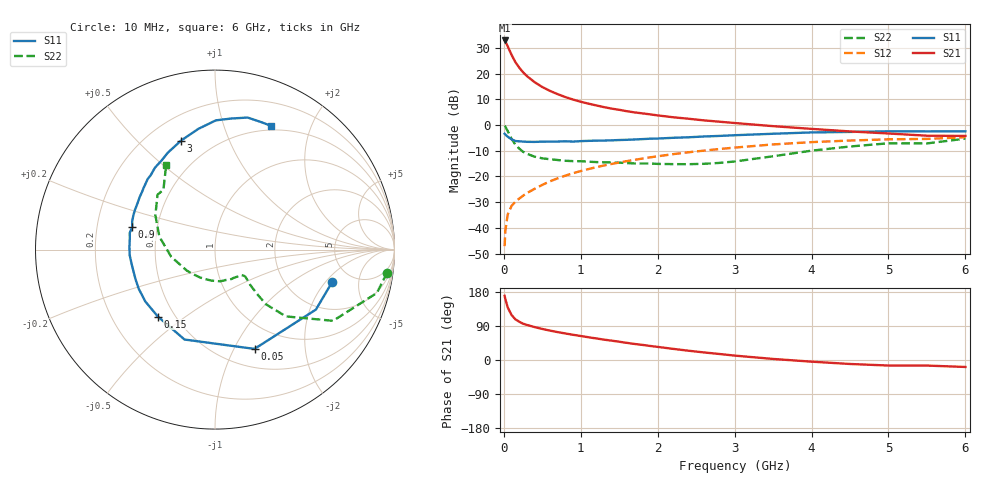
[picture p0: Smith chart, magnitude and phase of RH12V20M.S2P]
! SIEMENS Small Signal Semiconductors
! BFR106
! Si NPN RF Bipolar Junction Transistor in SOT23
! VCE = 12 V  IC = 20 mA
! Common Emitter S-Parameters:  August  1996
# GHz  S  MA  R  50
!  f  S11  S21  S12  S22
! GHz  MAG  ANG  MAG  ANG  MAG  ANG  MAG  ANG
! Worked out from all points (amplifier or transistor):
!   36 points, 10 MHz to 6 GHz, reference 50 ohm
!   highest |S21| = 33.0 dB at 10 MHz (marker M1)
!   |S21| within 3 dB of that: start of sweep to 60.87 MHz
!   unconditionally stable (mu >= 1): 386.3 MHz to 2.093 GHz
!   at 250 MHz: K = 0.86, MSG = 24.0 dB, |S12| = -27.5 dB
!   at 1.4 GHz: K = 1.08, MAG = 9.1 dB, |S12| = -15.1 dB
!   at 6 GHz: K = 0.98, MSG = 0.2 dB, |S12| = -4.7 dB
!   S11 on the Smith chart (normalised r, x): 10 MHz: 3.51, -2.36; 50 MHz: 0.71, -1.21; 150 MHz: 0.40, -0.40; 900 MHz: 0.36, +0.12; 3 GHz: 0.33, +0.68; 6 GHz: 0.45, +1.45
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0.01  0.677 -15.6  44.45 169.3  0.0044 83.1  0.9675 -7.6
0.02  0.6541 -30.7  42.46 160.8  0.0088 76.6  0.9336 -15.0
0.05  0.5954 -68.3  34.18 138.9  0.0182 63.7  0.7681 -31.1
0.1  0.529 -108.7  23.36 118.8  0.0267 55.2  0.5426 -43.3
0.15  0.4904 -130.5  16.85 107.3  0.0324 53.4  0.417 -47.0
0.2  0.4841 -143.3  13.17 101.0  0.0371 55.3  0.3495 -46.6
0.25  0.4778 -152.8  10.68 95.8  0.0422 58.0  0.3021 -45.7
0.3  0.4726 -159.6  8.995 92.5  0.0475 60.1  0.2764 -45.0
0.4  0.471 -169.4  6.851 86.9  0.0575 62.8  0.2429 -42.9
0.5  0.4763 -176.3  5.505 81.9  0.0686 64.8  0.2256 -41.7
0.6  0.477 178.1  4.631 77.6  0.0805 65.8  0.2167 -42.2
0.7  0.4785 172.8  4.002 73.6  0.0921 66.2  0.2092 -43.4
0.9  0.4779 164.8  3.14 66.5  0.1157 66.2  0.199 -45.8
1.1  0.4937 156.9  2.617 60.0  0.1395 65.2  0.1942 -51.4
1.3  0.5004 150.9  2.241 53.8  0.1636 63.9  0.1888 -56.8
1.6  0.5174 142.0  1.862 45.2  0.1992 61.3  0.1824 -68.0
2.2  0.566 126.2  1.422 29.4  0.2718 54.6  0.174 -95.2
3  0.6354 107.5  1.099 11.6  0.3651 43.9  0.1958 -143.3
3.5  0.6788 97.9  0.954 2.8  0.4206 36.6  0.2475 -170.8
4.5  0.7365 82.7  0.753 -10.5  0.5009 20.9  0.3833 150.1
5.5  0.7556 69.8  0.622 -14.7  0.5388 9.7  0.44 130.8
6  0.7566 65.7  0.616 -18.4  0.5817 2.0  0.5454 119.9
